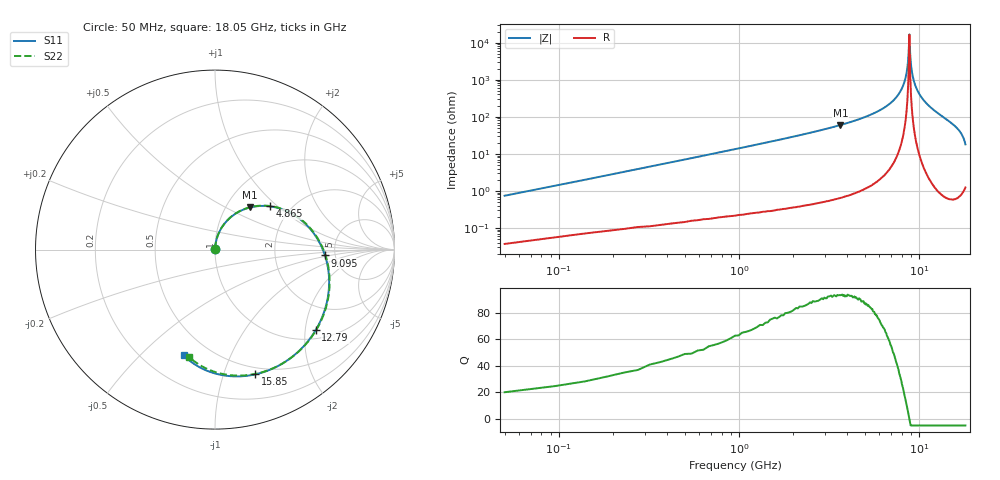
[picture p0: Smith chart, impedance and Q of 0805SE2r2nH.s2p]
! AVX Thin Film Operation		Date: May 2002
! Description: Accu-L® Series, Thin Film, SMD, RF Inductors
! Part Number: L08052R2CEWTR
! 50 MHz  -  18.05 GHz
! Serial Measurements
# mhz S db R 50
!	S11		S21		S12		S22
!	dB	Phase	dB	Phase	dB	Phase	dB	Phase
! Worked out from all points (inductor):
!   401 points, 50 MHz to 18.05 GHz, reference 50 ohm
!   read as 1/Y11, port 2 shorted: L = 2.26 nH near 140 MHz
!   highest Q = 93.1 at 3.65 GHz (marker M1), where L = 2.61 nH
!   self-resonance near 8.78 GHz
!   S11 on the Smith chart (normalised r, x): 50 MHz: 1.00, +0.01; 4.865 GHz: 1.58, +0.90; 9.095 GHz: 4.13, -0.43; 12.79 GHz: 1.24, -2.28; 15.85 GHz: 0.43, -1.28; 18.05 GHz: 0.36, -0.68
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50  -46.21 85.5  -0.00 -0.6  -0.00 -0.6  -46.21 85.5
185  -35.37 85.2  -0.01 -2.0  -0.01 -2.0  -35.37 85.2
320  -30.73 84.3  -0.01 -3.5  -0.01 -3.5  -30.73 84.3
545  -26.20 82.3  -0.02 -5.9  -0.02 -5.9  -26.20 82.3
815  -22.78 79.7  -0.04 -8.8  -0.04 -8.8  -22.78 79.7
1220  -19.36 75.5  -0.07 -13.1  -0.07 -13.1  -19.36 75.6
1715  -16.48 70.4  -0.12 -18.4  -0.12 -18.4  -16.48 70.6
3065  -11.71 56.4  -0.34 -32.6  -0.34 -32.6  -11.71 56.7
3650  -10.33 50.4  -0.46 -38.7  -0.46 -38.7  -10.33 50.7
4865  -8.17 38.1  -0.76 -51.0  -0.76 -51.0  -8.17 38.5
6080  -6.62 26.0  -1.12 -63.1  -1.12 -63.1  -6.62 26.5
7520  -5.28 12.0  -1.58 -77.2  -1.58 -77.2  -5.28 12.6
9050  -4.27 -2.6  -2.10 -91.8  -2.10 -91.8  -4.27 -1.8
9095  -4.24 -3.1  -2.12 -92.2  -2.12 -92.2  -4.24 -2.3
10580  -3.54 -17.1  -2.61 -106.3  -2.61 -106.3  -3.54 -16.2
12065  -3.05 -31.4  -3.06 -120.5  -3.06 -120.5  -3.05 -30.2
12785  -2.88 -38.5  -3.24 -127.6  -3.24 -127.6  -2.88 -37.2
13955  -2.69 -50.5  -3.46 -139.6  -3.46 -139.6  -2.69 -49.0
15080  -2.65 -62.8  -3.54 -152.0  -3.54 -152.0  -2.65 -61.1
15845  -2.73 -72.1  -3.46 -161.3  -3.46 -161.3  -2.73 -70.2
17060  -3.18 -89.1  -3.04 -178.5  -3.04 -178.5  -3.18 -86.7
18050  -4.23 -106.6  -2.31 163.6  -2.31 163.6  -4.22 -103.6
